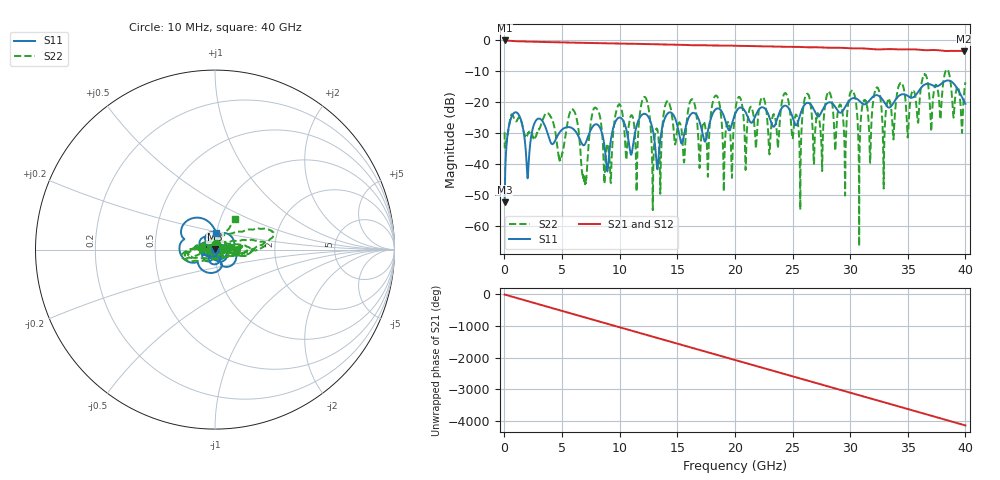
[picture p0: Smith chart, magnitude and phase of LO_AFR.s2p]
!Keysight Technologies,N5245B,MY57181321,A.13.80.12
!Automatic Fixture Removal (AFR)
!Date: Tuesday, May 12, 2020, 04:32:51
!S2P File: Measurements: S11,S21,S12,S22:
# MHz S  RI  R 50
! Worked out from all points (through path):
!   4000 points, 10 MHz to 40 GHz, reference 50 ohm
!   highest |S21| = -0.03 dB at 10 MHz (marker M1); lowest = -3.5 dB at 39.9 GHz (marker M2)
!   group delay of S21, straight-line fit = 287 ps
!   lowest |S11| = -52.4 dB at 10 MHz (marker M3), VSWR 1.00, Z = 50 + j0.239 ohm
!   |S11| at or under -10 dB: start of sweep to end of sweep
!   |S22| runs from -66.5 to -9.3 dB; largest |S21 - S12| = 1.5e-15
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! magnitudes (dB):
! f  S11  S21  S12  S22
! 10 MHz  -52.4  0.0  0.0  -29.7
! 880 MHz  -23.3  -0.3  -0.3  -25.6
! 2.01 GHz  -44.6  -0.4  -0.4  -30.4
! 4.87 GHz  -29.3  -0.6  -0.6  -38.5
! 5.95 GHz  -28.6  -0.7  -0.7  -22.4
! 6.68 GHz  -33.1  -0.8  -0.8  -40.6
! 7.88 GHz  -27.2  -0.9  -0.9  -21.7
! 8.74 GHz  -36.0  -0.9  -0.9  -40.9
! 9.93 GHz  -25.0  -1.1  -1.1  -20.7
! 11.48 GHz  -27.5  -1.1  -1.1  -46.6
! 12.13 GHz  -23.7  -1.2  -1.2  -18.3
! 13.34 GHz  -39.4  -1.3  -1.3  -30.6
! 14.14 GHz  -23.7  -1.4  -1.4  -19.6
! 15.55 GHz  -31.2  -1.4  -1.4  -38.8
! 16.24 GHz  -23.6  -1.6  -1.6  -19.1
! 16.96 GHz  -26.6  -1.6  -1.6  -39.8
! 18.3 GHz  -22.4  -1.7  -1.7  -17.9
! 20.01 GHz  -23.9  -1.7  -1.7  -23.1
! 26.67 GHz  -21.2  -2.2  -2.2  -24.5
! 33.34 GHz  -21.7  -2.8  -2.8  -19.2
! 39.9 GHz  -19.8  -3.5  -3.5  -16.7
! 40 GHz  -20.5  -3.4  -3.4  -13.5
